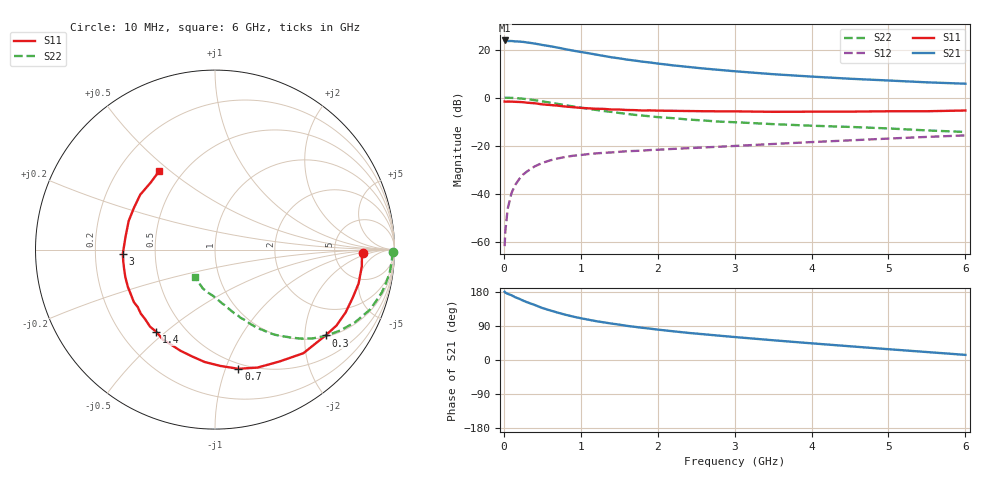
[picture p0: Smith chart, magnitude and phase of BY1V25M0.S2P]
! SIEMENS Small Signal Semiconductors
! BFY420
! Si NPN RF SIEGET Grounded Emitter Transistor in MICRO-X
! VCE = 1.25 V  IC = 5 mA
! Common Emitter S-Parameters:  October  1996
# GHz  S  MA  R  50
!  f  S11  S21  S12  S22
! GHz  MAG  ANG  MAG  ANG  MAG  ANG  MAG  ANG
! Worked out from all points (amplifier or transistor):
!   36 points, 10 MHz to 6 GHz, reference 50 ohm
!   highest |S21| = 23.8 dB at 10 MHz (marker M1)
!   |S21| within 3 dB of that: start of sweep to 704.1 MHz
!   unconditionally stable (mu >= 1): 3.096 GHz to end of sweep
!   at 250 MHz: K = 0.11, MSG = 27.6 dB, |S12| = -32.1 dB
!   at 1.4 GHz: K = 0.55, MSG = 19.8 dB, |S12| = -22.9 dB
!   at 6 GHz: K = 1.16, MAG = 8.3 dB, |S12| = -15.8 dB
!   S11 on the Smith chart (normalised r, x): 10 MHz: 10, -1; 300 MHz: 1.04, -2.55; 700 MHz: 0.45, -1.11; 1.4 GHz: 0.35, -0.47; 3 GHz: 0.32, -0.02; 6 GHz: 0.37, +0.46
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0.01  0.825 -1.5  15.44 180.0  0.0008 111.6  0.9894 -0.7
0.02  0.8196 -2.9  15.24 177.7  0.0017 92.5  0.9882 -1.4
0.05  0.8233 -6.5  15.04 174.7  0.0048 85.5  0.9871 -3.6
0.1  0.8221 -13.3  15.02 171.0  0.0103 84.6  0.9818 -7.4
0.15  0.8127 -19.4  14.77 165.3  0.0153 79.1  0.9709 -11.0
0.2  0.8076 -25.7  14.65 161.6  0.02 77.5  0.9598 -14.4
0.25  0.7982 -32.0  14.41 156.8  0.0248 72.9  0.941 -18.0
0.3  0.7802 -37.8  14.03 152.6  0.0287 70.4  0.9249 -21.3
0.4  0.7589 -49.5  13.31 145.3  0.0367 64.8  0.88 -27.3
0.5  0.7197 -60.0  12.44 137.2  0.0433 60.2  0.8314 -32.8
0.6  0.6986 -70.2  11.72 131.0  0.049 55.6  0.7831 -37.8
0.7  0.6767 -78.9  10.96 125.0  0.0537 52.1  0.7373 -42.1
0.9  0.629 -95.2  9.477 114.5  0.0612 46.0  0.6511 -48.9
1.1  0.5953 -109.0  8.374 106.3  0.0663 42.1  0.5809 -54.8
1.4  0.5626 -125.5  6.878 96.1  0.0718 38.0  0.5013 -61.2
1.8  0.5363 -143.4  5.593 85.0  0.0782 35.2  0.4208 -67.6
2.2  0.5279 -156.9  4.671 75.8  0.0851 33.2  0.371 -73.1
3  0.5144 -177.4  3.524 60.6  0.0979 31.5  0.3058 -81.8
3.5  0.5035 171.7  3.061 52.1  0.1076 30.0  0.2791 -87.0
4.5  0.5081 152.7  2.461 36.2  0.1281 25.9  0.244 -98.6
5.5  0.5177 133.8  2.071 21.0  0.1511 20.1  0.2061 -115.6
6  0.5361 125.6  1.938 13.5  0.1625 16.7  0.1915 -126.6
